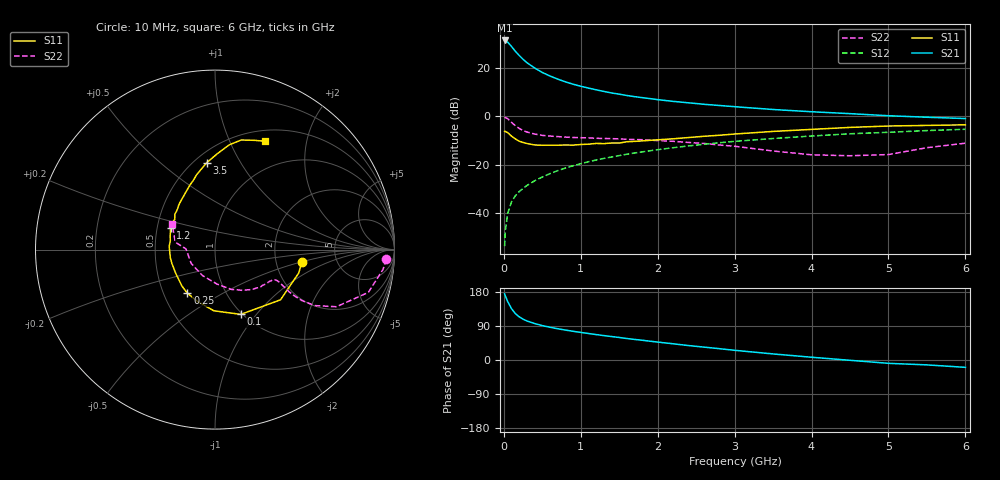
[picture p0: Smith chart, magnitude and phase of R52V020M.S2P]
! SIEMENS Small Signal Semiconductors
! BFR183
! Si NPN RF Bipolar Junction Transistor in SOT23
! VCE = 2 V  IC = 20 mA
! Common Emitter S-Parameters:  May  1996
# GHz  S  MA  R  50
!  f  S11  S21  S12  S22
! GHz  MAG  ANG  MAG  ANG  MAG  ANG  MAG  ANG
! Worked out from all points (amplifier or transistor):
!   36 points, 10 MHz to 6 GHz, reference 50 ohm
!   highest |S21| = 31.2 dB at 10 MHz (marker M1)
!   |S21| within 3 dB of that: start of sweep to 113 MHz
!   unconditionally stable (mu >= 1): 496.3 MHz to 2.406 GHz
!   at 250 MHz: K = 0.82, MSG = 26.6 dB, |S12| = -29.8 dB
!   at 1.4 GHz: K = 1.05, MAG = 11.8 dB, |S12| = -16.8 dB
!   at 6 GHz: K = 0.91, MSG = 2.2 dB, |S12| = -5.4 dB
!   S11 on the Smith chart (normalised r, x): 10 MHz: 2.81, -0.51; 100 MHz: 0.98, -0.84; 250 MHz: 0.66, -0.35; 1.2 GHz: 0.59, +0.15; 3.5 GHz: 0.57, +0.73; 6 GHz: 0.63, +1.37
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0.01  0.4886 -8.1  36.43 174.5  0.0021 83.6  0.9558 -3.2
0.02  0.4845 -15.6  36.1 168.9  0.0044 82.6  0.9428 -6.7
0.05  0.4598 -37.5  33.67 154.2  0.0099 74.0  0.8869 -15.6
0.1  0.3883 -68.3  27.36 135.4  0.0173 70.1  0.7476 -25.2
0.15  0.341 -91.1  21.8 122.3  0.023 67.8  0.6374 -29.3
0.2  0.3057 -107.8  17.84 113.9  0.028 67.2  0.5598 -30.4
0.25  0.2878 -122.2  14.87 107.7  0.0325 68.0  0.5067 -30.2
0.3  0.2742 -132.3  12.72 103.0  0.0374 68.8  0.4734 -29.6
0.4  0.2557 -148.8  9.863 96.3  0.0467 69.5  0.4295 -28.1
0.5  0.2523 -161.4  7.976 90.8  0.0559 71.1  0.4034 -27.0
0.6  0.253 -169.8  6.738 86.4  0.0656 71.1  0.39 -26.6
0.7  0.2526 -178.1  5.827 82.5  0.0756 71.2  0.3806 -26.5
0.8  0.2558 175.9  5.116 79.0  0.0854 70.5  0.3717 -26.8
0.9  0.2537 168.8  4.57 75.8  0.0954 70.3  0.3651 -27.2
1.1  0.2655 159.3  3.803 70.0  0.1154 69.1  0.3569 -29.3
1.2  0.2753 154.0  3.507 67.1  0.1252 68.6  0.3512 -30.3
1.6  0.2984 138.4  2.672 56.7  0.1648 64.5  0.3345 -36.0
2.2  0.3426 121.3  2.024 42.8  0.2244 58.1  0.3045 -46.9
3.5  0.4867 95.4  1.376 16.0  0.3472 41.4  0.1919 -86.9
4.5  0.5886 82.3  1.13 -0.8  0.4353 28.4  0.1533 -149.7
5.5  0.6467 70.3  0.953 -12.9  0.5063 16.5  0.225 169.4
6  0.665 65.2  0.896 -19.4  0.5386 8.8  0.2782 149.1
